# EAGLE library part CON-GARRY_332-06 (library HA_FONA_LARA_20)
6 Pin - 2mm Dual Row Source: www.mpe-connector.de / garry_shortform_2012.pdf
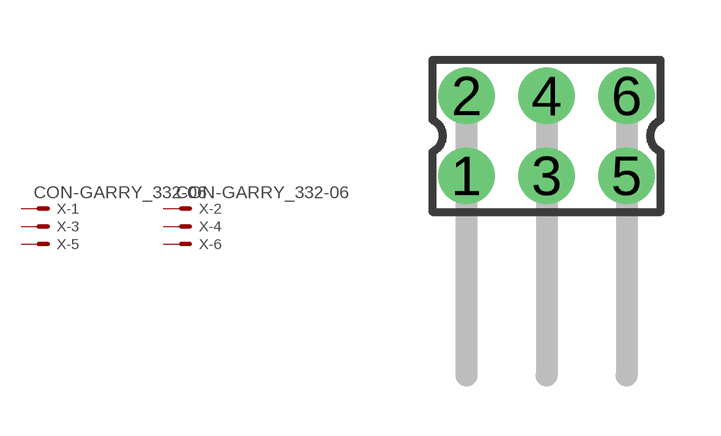
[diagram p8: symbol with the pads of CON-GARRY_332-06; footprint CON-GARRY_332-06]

Designator prefix X; gates -1=CON-GARRY_MV -2=CON-GARRY_MV -3=CON-GARRY_M -4=CON-GARRY_M -5=CON-GARRY_M -6=CON-GARRY_M

## CON-GARRY_332-06  [CON-GARRY_332-06]
1  -1:S  pas
2  -2:S  pas
3  -3:S  pas
4  -4:S  pas
5  -5:S  pas
6  -6:S  pas

## Footprint CON-GARRY_332-06 (pad centres in mm)
6 Pin - 2mm Dual Row Source: www.mpe-connector.de / garry_shortform_2012.pdf
drill 0.9 pad 1.27: 1 -2,-1; 2 -2,1; 3 0,-1; 4 0,1; 5 2,-1; 6 2,1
